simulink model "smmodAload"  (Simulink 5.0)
settings: Solver=ode45  StartTime=0.0  StopTime=5  MaxStep=1e-3  RelTol=1e-4  AbsTol=1e-4
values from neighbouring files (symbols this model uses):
  Bm = 0.10    (= 0.1)    [IMabc2.m]    (also in imabcparam.m = 0.01; IMabcrun0.m = 0.01; IMabcrun1.m = 0.001; IMcur0.m = 1e-06)
  H = 0.60    (= 0.6)    [IMabc2.m]    (also in IMcur0.m = 0.3; imdef0vec.m = 0.3; imdef1vec.m = 0.3; imdef2vec.m = 0.3)
  n0 = 0.98    [imdef0vec.m]    (also in imdef1vec.m = 0.978; imdef2vec.m; imdefrotflux.m; imdefSIvec1.m = 0.95)
  Ra = .95    (= 0.95)    [altwdgs.m]    (also in Ccurverun.m = 0.018)
  tc = abs(fco)    [im3phase.m]
  Te0 = 0.75/wo*p*(Is*conj(Is)*Req)    [imdefSIvec1.m]
  V = [Vas 0 0].'    [Actac.m]    (also in acttrcalc1.m = str2num(get(h,'string')); im3d.m = eval(get(hVs,'String')); IMabc2.m = [vas vbs vcs 0 0 0]'; IMabcf0.m = [vas vbs vcs 0 0 0]')
  wo = 2*pi*freq0    [calc0.m]    (also in IMabc2.m = 376.991118431; imabcparam.m = 376.991118431; IMabcrun0.m = 376.991118431; IMabcrun1.m = 376.991118431)
undefined symbols (not defined in the file or in its folder): delta0, fk0, L_1, phif0, Rf, Rkd, Rkq, vf0
libraries: simulink x1

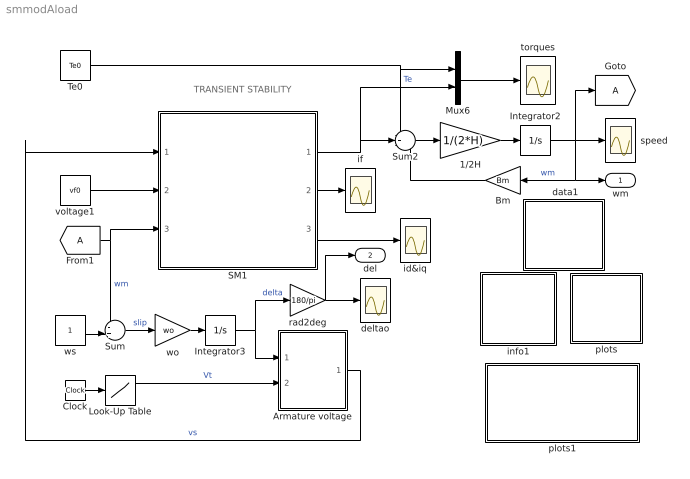
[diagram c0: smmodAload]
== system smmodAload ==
  note: TRANSIENT STABILITY
  " data1" : Subsystem
  1/2H : Gain  Gain=1/(2*H)
  Armature voltage : Subsystem
  Bm : Gain  Orientation=left  Gain=Bm
  Clock : Clock
  Integrator2 : Integrator  InitialCondition=n0
  Integrator3 : Integrator  InitialCondition=delta0
  Look-Up Table : Lookup  InputValues=[0 0.5 0.5 0.5+tc 0.5+tc 3]  OutputValues=[V V 0 0 V V]
  Mux6 : Mux  Inputs=2
  SM1 : Subsystem
  Sum : Sum  Inputs=-+|
  Sum2 : Sum  Inputs=-+-
  Te0 : Constant  Value=Te0
  deltao : Scope
  id&iq : Scope
  if : Scope
  info1 : Subsystem
  plots : Subsystem
  plots1 : Subsystem
  rad2deg : Gain  Gain=180/pi
  speed : Scope
  torques : Scope
  voltage1 : Constant  Value=vf0
  wo : Gain  Gain=wo
  ws : Constant
  wm : Outport
  del : Outport  Port=2
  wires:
  Mux6/1 -> torques/1
  voltage1/1 -> SM1/2(vf)
  SM1/2(if) -> if/1
  Sum2/1 -> 1/2H/1
  1/2H/1 -> Integrator2/1
  SM1/1(Te) -> Sum2/2, Mux6/2  "Te"
  Bm/1 -> Sum2/3
  Integrator2/1 -> speed/1, [A], Bm/1, wm/1  "wm"
  Te0/1 -> Mux6/1, Sum2/1
  ws/1 -> Sum/2
  Sum/1 -> wo/1  "slip"
  wo/1 -> Integrator3/1
  Armature voltage/1(vs) -> SM1/1(vs)  "vs"
  Integrator3/1 -> Armature voltage/1(delta), rad2deg/1  "delta"
  SM1/3(ia) -> id&iq/1
  rad2deg/1 -> deltao/1, del/1
  Clock/1 -> Look-Up Table/1
  Look-Up Table/1 -> Armature voltage/2(Vt)  "Vt"
  [A] -> Sum/1, SM1/3(wm)  "wm"

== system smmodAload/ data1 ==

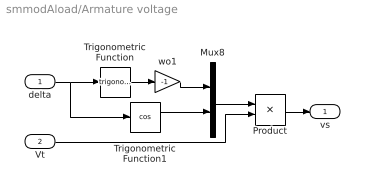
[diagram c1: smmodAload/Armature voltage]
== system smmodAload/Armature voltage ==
  delta : Inport
  Vt : Inport  Port=2
  Mux8 : Mux  Inputs=2
  Product : Product
  Trigonometric Function : Trigonometry
  Trigonometric Function1 : Trigonometry  Operator=cos
  wo1 : Gain  Gain=-1
  vs : Outport
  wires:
  delta/1 -> Trigonometric Function/1, Trigonometric Function1/1
  Trigonometric Function/1 -> wo1/1
  Mux8/1 -> Product/1
  wo1/1 -> Mux8/1
  Trigonometric Function1/1 -> Mux8/2
  Product/1 -> vs/1
  Vt/1 -> Product/2

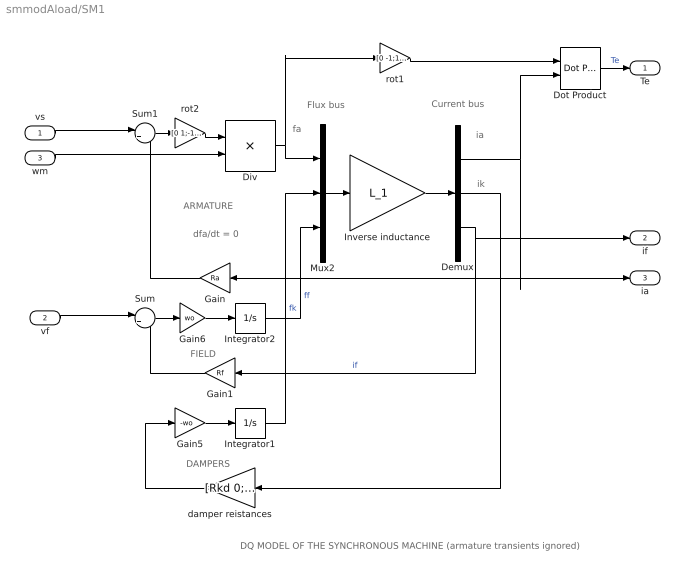
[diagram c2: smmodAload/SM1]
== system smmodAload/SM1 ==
  note: DAMPERS
  note: ARMATURE
  note: fa
  note: ia
  note: FIELD
  note: DQ MODEL OF THE SYNCHRONOUS MACHINE (armature transients ignored)
  note: Flux bus
  note: Current bus
  note: dfa/dt = 0
  note: ik
  vs : Inport
  vf : Inport  Port=2
  wm : Inport  Port=3
  Demux : Demux  Outputs=3
  Div : Product  Inputs=*/  Multiplication=Matrix(*)
  Dot Product : simulink/Math Operations/Dot Product
  Gain : Gain  Orientation=left  Gain=Ra
  Gain1 : Gain  Orientation=left  Gain=Rf
  Gain5 : Gain  Gain=-wo
  Gain6 : Gain  Gain=wo
  Integrator1 : Integrator  InitialCondition=fk0
  Integrator2 : Integrator  InitialCondition=phif0
  Inverse inductance : Gain  Gain=L_1  Multiplication=Matrix(K*u)
  Mux2 : Mux  Inputs=3
  Sum : Sum  Inputs=|+-
  Sum1 : Sum  Inputs=|+-
  damper reistances : Gain  Orientation=left  Gain=[Rkd 0;0 Rkq]  Multiplication=Matrix(K*u)
  rot1 : Gain  Gain=[0 -1;1 0]  Multiplication=Matrix(K*u)
  rot2 : Gain  Gain=[0 1;-1 0]  Multiplication=Matrix(K*u)
  Te : Outport
  if : Outport  Port=2
  ia : Outport  Port=3
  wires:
  Gain5/1 -> Integrator1/1
  damper reistances/1 -> Gain5/1
  Sum1/1 -> rot2/1
  Gain/1 -> Sum1/2
  Gain6/1 -> Integrator2/1
  Sum/1 -> Gain6/1
  vf/1 -> Sum/1
  Gain1/1 -> Sum/2
  rot1/1 -> Dot Product/1
  Demux/1 -> Gain/1, ia/1, Dot Product/2
  Dot Product/1 -> Te/1  "Te"
  Mux2/1 -> Inverse inductance/1
  Inverse inductance/1 -> Demux/1
  Integrator1/1 -> Mux2/2  "fk"
  Integrator2/1 -> Mux2/3  "ff"
  Demux/2 -> damper reistances/1
  Demux/3 -> if/1, Gain1/1  "if"
  vs/1 -> Sum1/1
  Div/1 -> Mux2/1, rot1/1
  rot2/1 -> Div/1
  wm/1 -> Div/2

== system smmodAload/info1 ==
  note: Synchronous machine transients
  note: This demonstration illustrates the dynamics of a synchronous machine following the sudden application and removal of a three-phase short circuit at the terminals. To modify the parameters and loading conditions, click the yellow block. Start the simulation. Four models of the synchronous machine are provided: 1) A complete model (5th-order) 2) Armature transients ignored by setting dfa/dt=0 (3rd-order) 3) Both armature transients and damper effects are neglected (1st-order) 4) Constant field flux linkage (zero-order)

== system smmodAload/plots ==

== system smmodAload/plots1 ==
